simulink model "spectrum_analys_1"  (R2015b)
settings: Solver=FixedStepAuto  StartTime=0.0  StopTime=10.0  RelTol=1e-3
undefined symbols (not defined in the file or in its folder): fir1
libraries: dspstat3 x2, simulink x1

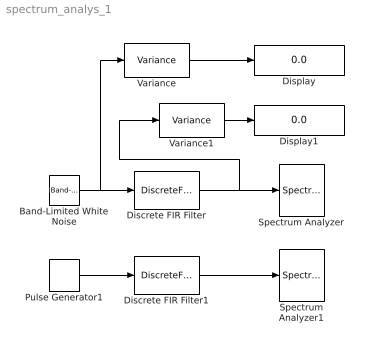
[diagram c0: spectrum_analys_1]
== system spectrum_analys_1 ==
  Band-Limited White Noise : simulink/Sources/Band-Limited White Noise  Cov=1/1000  Ts=1/1000  seed=[23341]
  Discrete FIR Filter : DiscreteFir  Coefficients=fir1(256, 0.4)
  Discrete FIR Filter1 : DiscreteFir  Coefficients=fir1(256, 0.4)  SampleTime=1/1000
  Display : Display
  Display1 : Display
  Pulse Generator1 : DiscretePulseGenerator  Period=50  PulseWidth=25  SampleTime=1/1000
  Spectrum Analyzer : SpectrumAnalyzer
  Spectrum Analyzer1 : SpectrumAnalyzer
  Variance : dspstat3/Variance  run=on  reset_popup=None  InputProcessing=Columns as channels (frame based)  directionMode=Each column  dimension=1  roiEnable=off  roiType=Rectangles  roiPortion=Entire ROI  roiOutput=Individual statistics for each ROI  roiFlag=off  roundingMode=Floor  overflowMode=off
  Variance1 : dspstat3/Variance  run=on  reset_popup=None  InputProcessing=Columns as channels (frame based)  directionMode=Each column  dimension=1  roiEnable=off  roiType=Rectangles  roiPortion=Entire ROI  roiOutput=Individual statistics for each ROI  roiFlag=off  roundingMode=Floor  overflowMode=off
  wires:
  Band-Limited White Noise/1 -> Variance/1, Discrete FIR Filter/1
  Discrete FIR Filter/1 -> Variance1/1, Spectrum Analyzer/1
  Variance/1 -> Display/1
  Variance1/1 -> Display1/1
  Pulse Generator1/1 -> Discrete FIR Filter1/1
  Discrete FIR Filter1/1 -> Spectrum Analyzer1/1
